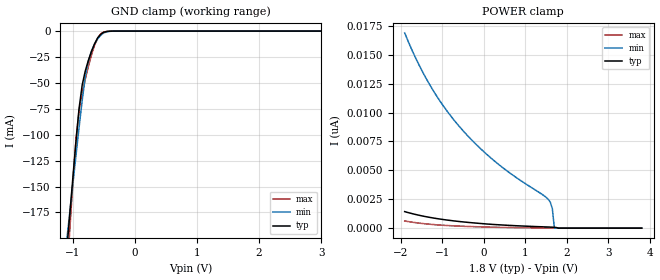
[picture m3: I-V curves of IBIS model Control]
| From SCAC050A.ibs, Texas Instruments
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[Model]   Control
Model_type   Input
|Signals   OS, OE
Vinh = 1.105V
Vinl = 0.665V
|   typ   min   max
C_comp   1.13pF   NA   NA
|   typ   min   max
[Temperature Range]   40   105   0
[Voltage range]   1.8   1.7   1.9
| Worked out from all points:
|   GND clamp passes 1 mA (typ) near -0.50 V on its own axis
[Power Clamp]
|   Voltage   I(typ)   I(min)   I(max)
-1.9V     1.432nA    16.9nA     623.1pA
-1.65V    1.195nA    14.83nA    480.5pA
-1.4V     1.001nA    13.06nA    374.3pA
-1.1V     814.2pA    11.26nA    281pA
-800mV    664.5pA    9.748nA    213.7pA
-350mV    490.5pA    7.861nA    143.9pA
150mV     341.1pA    6.144nA    87.33pA
1.55V     98.37pA    2.506nA    15.89pA
1.6V      91.25pA    2.261nA    14.16pA
1.65V     83.28pA    1.687nA    12.44pA
1.7V      73.05pA    0A         10.69pA
3.8V      0A         0A         0A
[GND Clamp]
|   Voltage   I(typ)   I(min)   I(max)
-1.9V     -784.2mA   -642.1mA   -981.4mA
-1.1V     -212.8mA   -202.5mA   -238.6mA
-1.05V    -177.1mA   -175.1mA   -192.3mA
-950mV    -106.5mA   -120.2mA   -104.7mA
-900mV    -74.68mA   -93.04mA   -76.27mA
-850mV    -52.07mA   -66.94mA   -59.64mA
-800mV    -38.45mA   -44.46mA   -46.28mA
-750mV    -28.28mA   -28.92mA   -34.05mA
-700mV    -19.55mA   -19.28mA   -22.99mA
-600mV    -6.54mA    -7.452mA   -6.745mA
-500mV    -1.069mA   -1.715mA   -861.5uA
3.8V      0A         0A         0A
